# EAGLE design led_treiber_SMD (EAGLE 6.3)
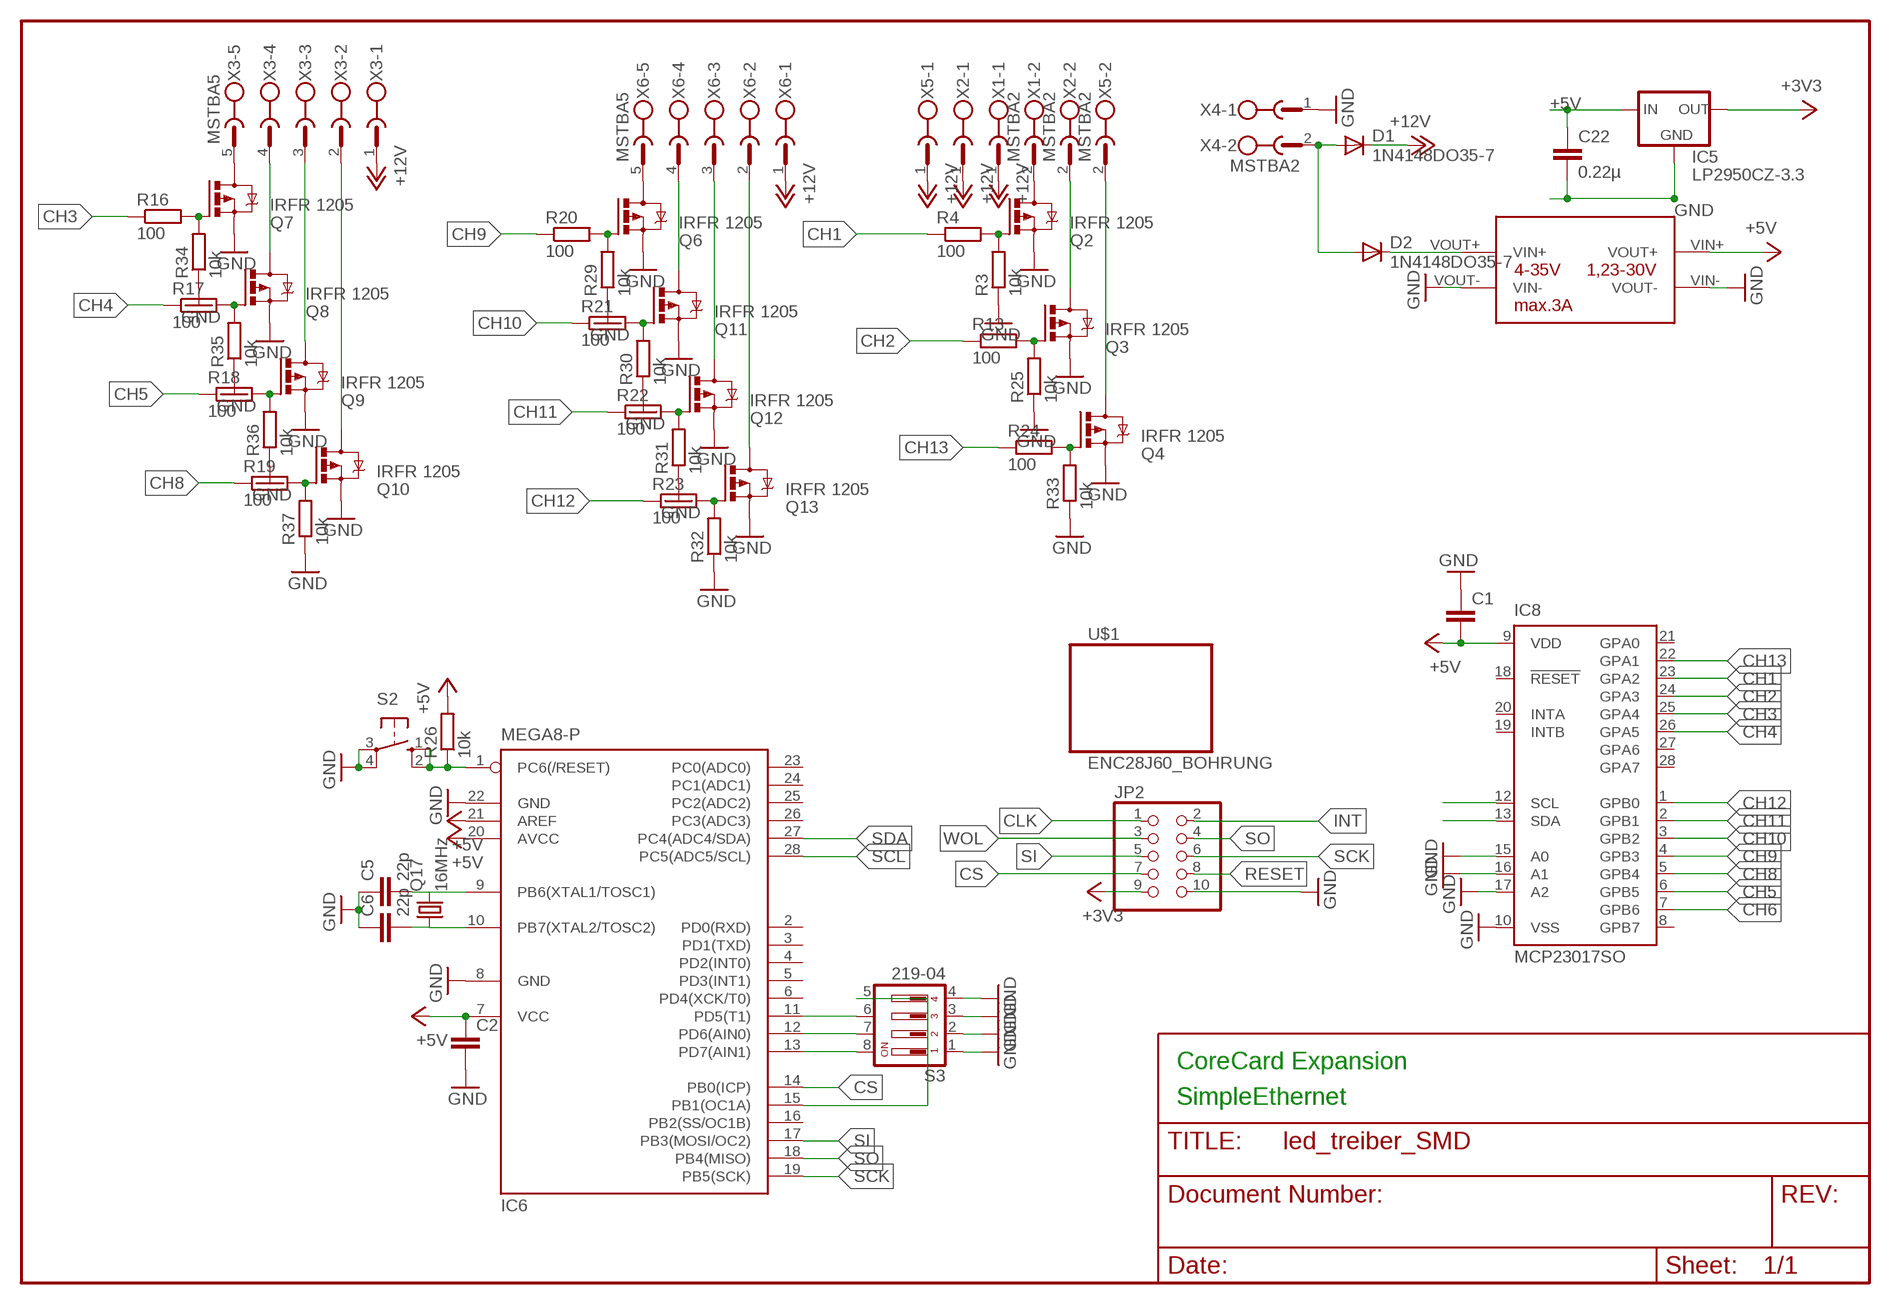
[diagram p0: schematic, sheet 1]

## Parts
C1  C-EUC0805  [C0805]
C2  C-EUC0805  [C0805]
C5  22p  C-EU025-025X050  [C025-025X050]
C6  22p  C-EU025-025X050  [C025-025X050]
C22  0.22µ  C-EUC0603  [C0603]
D1  1N4148DO35-7  [DO35-7]
D2  1N4148DO35-7  [DO35-7]
IC5  LP2950CZ-3.3  [TO92]
IC6  MEGA8-P  [DIL28-3]
IC8  MCP23017SO  [SO28W]
JP2  PINHD-2X5  [2X05]
Q2  IRFR 1205  IRFR5305  [D-PAK_TO252AA]
Q3  IRFR 1205  IRFR5305  [D-PAK_TO252AA]
Q4  IRFR 1205  IRFR5305  [D-PAK_TO252AA]
Q6  IRFR 1205  IRFR5305  [D-PAK_TO252AA]
Q7  IRFR 1205  IRFR5305  [D-PAK_TO252AA]
Q8  IRFR 1205  IRFR5305  [D-PAK_TO252AA]
Q9  IRFR 1205  IRFR5305  [D-PAK_TO252AA]
Q10  IRFR 1205  IRFR5305  [D-PAK_TO252AA]
Q11  IRFR 1205  IRFR5305  [D-PAK_TO252AA]
Q12  IRFR 1205  IRFR5305  [D-PAK_TO252AA]
Q13  IRFR 1205  IRFR5305  [D-PAK_TO252AA]
Q17  16MHz  CRYSTALHC49S  [HC49/S]
R3  10k  R-EU_M0805  [M0805]
R4  100  R-EU_R0805  [R0805]
R13  100  R-EU_M0805  [M0805]
R16  100  R-EU_M0805  [M0805]
R17  100  R-EU_M0805  [M0805]
R18  100  R-EU_M0805  [M0805]
R19  100  R-EU_M0805  [M0805]
R20  100  R-EU_R0805  [R0805]
R21  100  R-EU_R0805  [R0805]
R22  100  R-EU_R0805  [R0805]
R23  100  R-EU_M0805  [M0805]
R24  100  R-EU_M0805  [M0805]
R25  10k  R-EU_R0805  [R0805]
R26  10k  R-EU_M0805  [M0805]
R29  10k  R-EU_R0805  [R0805]
R30  10k  R-EU_R0805  [R0805]
R31  10k  R-EU_R0805  [R0805]
R32  10k  R-EU_M0805  [M0805]
R33  10k  R-EU_M0805  [M0805]
R34  10k  R-EU_M0805  [M0805]
R35  10k  R-EU_M0805  [M0805]
R36  10k  R-EU_M0805  [M0805]
R37  10k  R-EU_M0805  [M0805]
S2  10-XX  [B3F-10XX]
S3  219-04  [CTS-219-04]
U$1  ENC28J60_BOHRUNG  [ENC28J60_BOHRUNG]
U$2  SCHALTREGLER  [SCHALTREGLER_PLATINE]
X1  MSTBA2  [MSTBA2]
X2  MSTBA2  [MSTBA2]
X3  MSTBA5  [MSTBA5]
X4  MSTBA2  [MSTBA2]
X5  MSTBA2  [MSTBA2]
X6  MSTBA5  [MSTBA5]

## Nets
+3V3: IC5.1(OUT) JP2.9
+5V: C1.2 C2.1 C22.1 IC5.3(IN) IC6.7(VCC) IC6.20(AVCC) IC6.21(AREF) IC8.9(VDD) R26.2 U$2.VIN+(VOUT+)
+12V: D1.C X1.1 X2.1 X3.1 X5.1 X6.1
CH1: IC8.23(GPA2) R4.1
CH2: IC8.24(GPA3) R13.1
CH3: IC8.25(GPA4) R16.1
CH4: IC8.26(GPA5) R17.1
CH5: IC8.6(GPB5) R18.1
CH6: IC8.7(GPB6)
CH8: IC8.5(GPB4) R19.1
CH9: IC8.4(GPB3) R20.1
CH10: IC8.3(GPB2) R21.1
CH11: IC8.2(GPB1) R22.1
CH12: IC8.1(GPB0) R23.1
CH13: IC8.22(GPA1) R24.1
CLK: JP2.1
CS: IC6.14(PB0(ICP)) JP2.7
GND: C1.1 C2.2 C5.1 C6.1 C22.2 IC5.2(GND) IC6.8(GND) IC6.22(GND) IC8.10(VSS) IC8.15(A0) IC8.16(A1) IC8.17(A2) JP2.10 Q2.3(S) Q3.3(S) Q4.3(S) Q6.3(S) Q7.3(S) Q8.3(S) Q9.3(S) Q10.3(S) Q11.3(S) Q12.3(S) Q13.3(S) R3.1 R25.1 R29.1 R30.1 R31.1 R32.1 R33.1 R34.1 R35.1 R36.1 R37.1 S2.3(P) S2.4(P1) S3.1 S3.2 S3.3 S3.4 U$2.VIN-(VOUT-) U$2.VOUT-(VIN-) X4.1
INT: JP2.2
N$8: Q2.4(D) X1.2
N$11: Q6.4(D) X6.5
N$12: Q7.4(D) X3.5
N$15: Q2.1(G) R3.2 R4.2
N$19: Q3.1(G) R13.2 R25.2
N$20: Q4.4(D) X5.2
N$21: IC6.15(PB1(OC1A)) S3.5
N$22: Q7.1(G) R16.2 R34.2
N$23: Q8.1(G) R17.2 R35.2
N$24: Q9.1(G) R18.2 R36.2
N$25: Q10.1(G) R19.2 R37.2
N$26: Q6.1(G) R20.2 R29.2
N$27: Q11.1(G) R21.2 R30.2
N$28: Q12.1(G) R22.2 R31.2
N$29: Q13.1(G) R23.2 R32.2
N$30: Q4.1(G) R24.2 R33.2
N$31: D1.A D2.A X4.2
N$32: C5.2 IC6.9(PB6(XTAL1/TOSC1)) Q17.2
N$33: C6.2 IC6.10(PB7(XTAL2/TOSC2)) Q17.1
N$34: D2.C U$2.VOUT+(VIN+)
N$36: IC6.11(PD5(T1)) S3.6
N$37: IC6.12(PD6(AIN0)) S3.7
N$38: Q3.4(D) X2.2
N$41: IC6.13(PD7(AIN1)) S3.8
N$42: Q8.4(D) X3.4
N$43: Q9.4(D) X3.3
N$44: Q10.4(D) X3.2
N$46: Q11.4(D) X6.4
N$47: Q12.4(D) X6.3
N$48: Q13.4(D) X6.2
RESET: IC6.1(PC6(/RESET)) JP2.8 R26.1 S2.1(S) S2.2(S1)
SCK: IC6.19(PB5(SCK)) JP2.6
SCL: IC6.28(PC5(ADC5/SCL)) IC8.12(SCL)
SDA: IC6.27(PC4(ADC4/SDA)) IC8.13(SDA)
SI: IC6.17(PB3(MOSI/OC2)) JP2.5
SO: IC6.18(PB4(MISO)) JP2.4
WOL: JP2.3
Unconnected: IC6.2(PD0(RXD)) IC6.3(PD1(TXD)) IC6.4(PD2(INT0)) IC6.5(PD3(INT1)) IC6.6(PD4(XCK/T0)) IC6.16(PB2(SS/OC1B)) IC6.23(PC0(ADC0)) IC6.24(PC1(ADC1)) IC6.25(PC2(ADC2)) IC6.26(PC3(ADC3)) IC8.8(GPB7) IC8.18(!RESET) IC8.19(INTB) IC8.20(INTA) IC8.21(GPA0) IC8.27(GPA6) IC8.28(GPA7)

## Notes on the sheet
- CoreCard Expansion
- SimpleEthernet

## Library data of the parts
C1 C2 C5 C6 C22 = rcl:C-EU: CAPACITOR, European symbol
D1 D2 = diode:1N4148: DIODE
IC5 = v-reg:LP2950?*: Source: http://cache.national.com/ds/LP/LP2950.pdf
IC6 = atmel:MEGA8-P: MICROCONTROLLER 8 Kbytes FLASH, 1 kbytes SRAM, 512 bytes EEPROM, USART, 4-channel 10 bit ADC, 2-channel 8 bit ADC Pin compatible with Atmega48, ATMega88, ATMega168 Source: avr.lbr; OC_FARNELL: unknown; OC_NEWARK: unknown
IC8 = microchip:MCP23017: http://ww1.microchip.com/downloads/en/DeviceDoc/21952a.pdf Source: http://ww1.microchip.com/downloads/en/DeviceDoc/21952a.pdf; MF: MICROCHIP; MPN: MCP23017-E/SO; OC_FARNELL: 1332087; OC_NEWARK: 31K2958
JP2 = pinhead:PINHD-2X5: PIN HEADER
Q2-Q4 Q6-Q13 = transistor-power:IRF?5305: HEXFET Power MOSFET Source: http://www.irf.com/product-info/datasheets/data/irfr5305pbf.pdf
Q17 = crystal:CRYSTAL: CRYSTAL; OC_FARNELL: 1667008; OC_NEWARK: unknown
R3 R4 R13 R16-R26 R29-R37 = rcl:R-EU_: RESISTOR, European symbol
S2 = switch-omron:10-XX: OMRON SWITCH; MPN: B3F-1000; OC_FARNELL: 176432; OC_NEWARK: 36M3542
S3 = switch-dil:219-04*: Surface Mount DIP Switch Series 219 SMT CTS Electronic Components Sourc: www.ctscorp.com; OC_FARNELL: unknown; OC_NEWARK: unknown
U$1 = daniel:ENC28J60_BOHRUNG
U$2 = daniel:SCHALTREGLER
X1 X2 X4 X5 = con-phoenix-508:MSTBA2: PHOENIX; MF: FARNELL; MPN: 1757242; OC_FARNELL: 3705171; OC_NEWARK: 71C4161
X3 X6 = con-phoenix-508:MSTBA5: PHOENIX; MPN: 1757271; OC_FARNELL: 3705201; OC_NEWARK: 71C4164

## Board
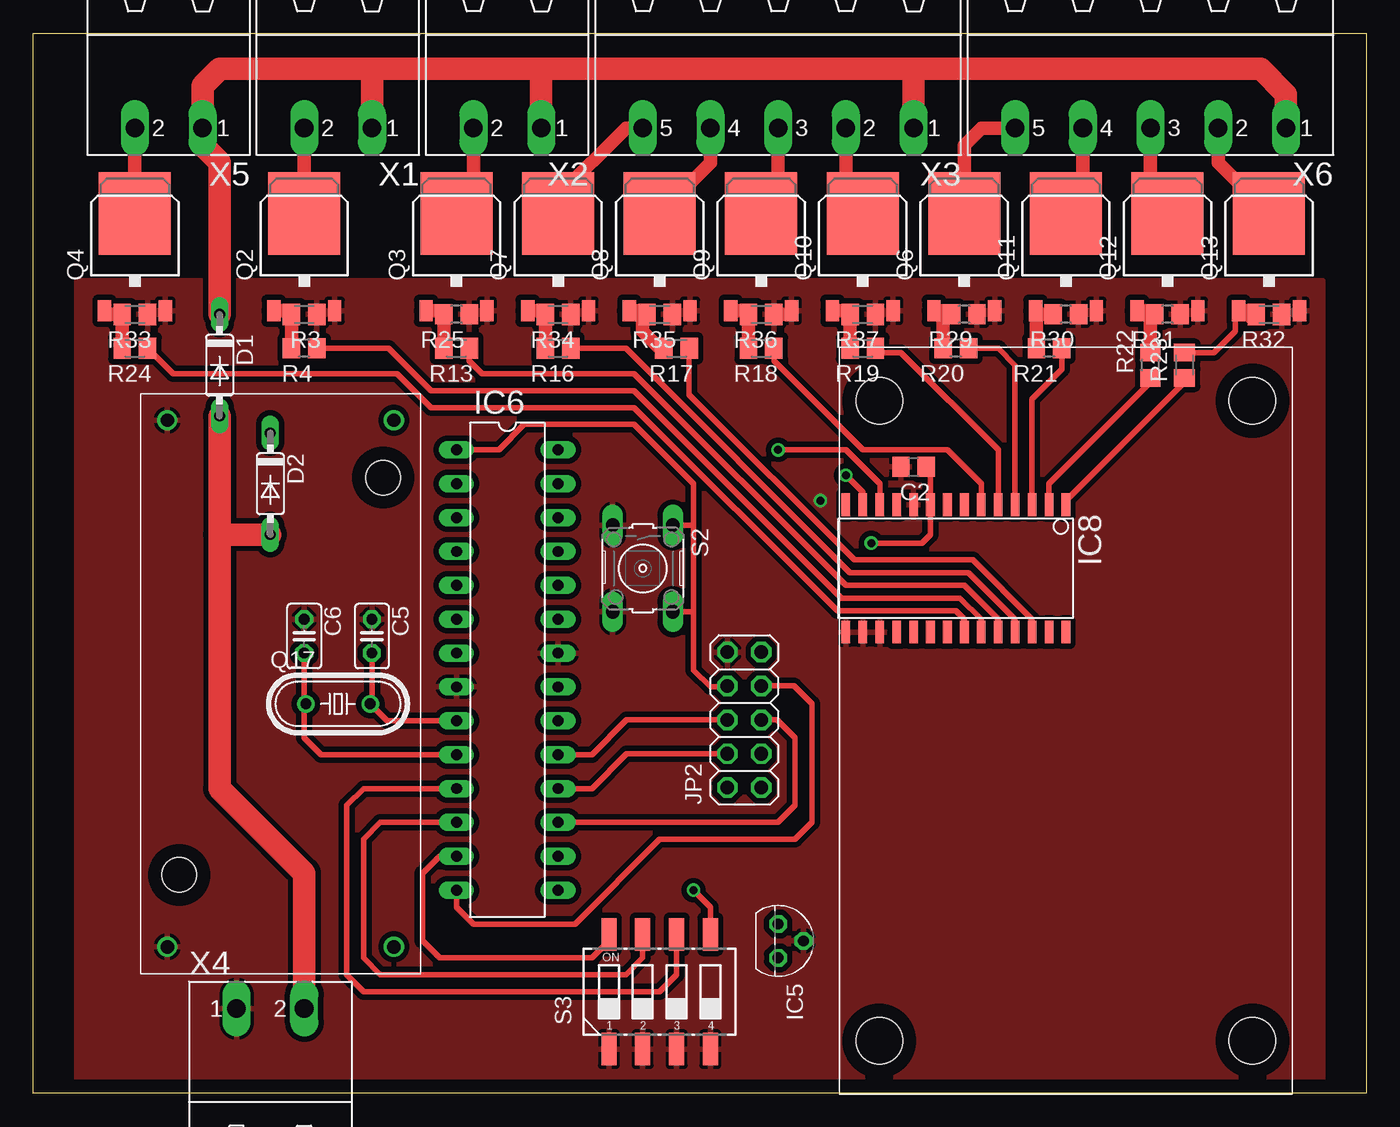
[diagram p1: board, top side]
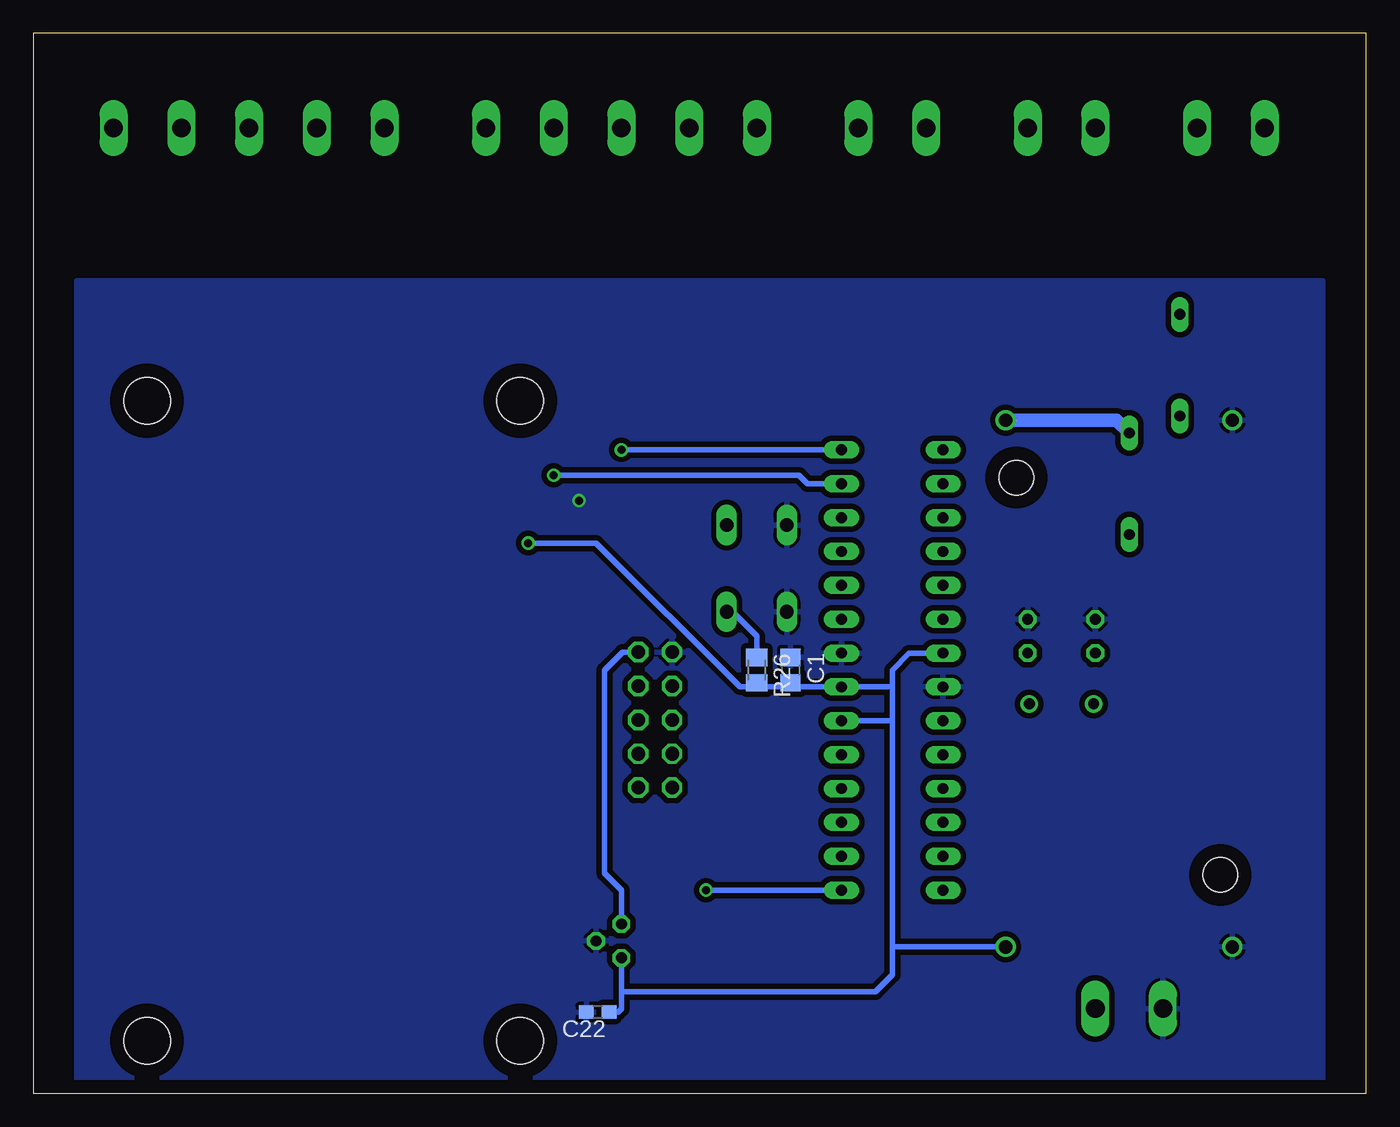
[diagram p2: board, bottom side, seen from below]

Size 100 x 79.5 mm. Coordinates in mm from the lower left corner, seen from the top.
Outline: 0,0 0,79.5 100,79.5 100,0 0,0
Copper layers (1*16): Top 0.035mm / dielectric 1.5mm / Bottom 0.035mm
Design rules "Bilex DRU": minimum track width 10mil, minimum drill 24mil, track to track 10mil, track to pad 10mil, pad to pad 10mil, via to via 10mil, smd to smd 10mil, copper to edge 40mil, drill to drill 8mil, minimum pad ring 10mil, minimum via ring 8mil, stop-mask expansion 4mil, vias tented up to drill 0mil, thermal gap 10mil

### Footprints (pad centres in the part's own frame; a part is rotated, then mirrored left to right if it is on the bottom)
C0805 = smd 1.3 x 1.5: 1 -0.95,0; 2 0.95,0
C025-025X050 = drill 0.813 octagon: 1 -1.27,0; 2 1.27,0
C0603 = smd 1.1 x 1: 1 -0.85,0; 2 0.85,0
DO35-7 = drill 0.813 long: A 3.81,0; C -3.81,0
TO92 = drill 0.813 octagon: 1 -1.27,0; 2 0,1.905; 3 1.27,0
DIL28-3 = drill 0.813 long: 1 -16.51,-3.81; 2 -13.97,-3.81; 3 -11.43,-3.81; 4 -8.89,-3.81; 5 -6.35,-3.81; 6 -3.81,-3.81; 7 -1.27,-3.81; 8 1.27,-3.81; 9 3.81,-3.81; 10 6.35,-3.81; 11 8.89,-3.81; 12 11.43,-3.81; 13 13.97,-3.81; 14 16.51,-3.81; 15 16.51,3.81; 16 13.97,3.81; 17 11.43,3.81; 18 8.89,3.81; 19 6.35,3.81; 20 3.81,3.81; 21 1.27,3.81; 22 -1.27,3.81; 23 -3.81,3.81; 24 -6.35,3.81; 25 -8.89,3.81; 26 -11.43,3.81; 27 -13.97,3.81; 28 -16.51,3.81
SO28W = smd 0.65 x 1.7: 1 -7.62,-4.78; 2 -6.35,-4.78; 3 -5.08,-4.78; 4 -3.81,-4.78; 5 -2.54,-4.78; 6 -1.27,-4.78; 7 0,-4.78; 8 1.27,-4.78; 9 2.54,-4.78; 10 3.81,-4.78; 11 5.08,-4.78; 12 6.35,-4.78; 13 7.62,-4.78; 14 8.89,-4.78; 15 8.89,4.78; 16 7.62,4.78; 17 6.35,4.78; 18 5.08,4.78; 19 3.81,4.78; 20 2.54,4.78; 21 1.27,4.78; 22 0,4.78; 23 -1.27,4.78; 24 -2.54,4.78; 25 -3.81,4.78; 26 -5.08,4.78; 27 -6.35,4.78; 28 -7.62,4.78
2X05 = drill 1.016 octagon: 1 -5.08,-1.27; 2 -5.08,1.27; 3 -2.54,-1.27; 4 -2.54,1.27; 5 0,-1.27; 6 0,1.27; 7 2.54,-1.27; 8 2.54,1.27; 9 5.08,-1.27; 10 5.08,1.27
D-PAK_TO252AA = smd 1 x 1.6: 1 -2.28,-4.8; 3 2.28,-4.8 | smd 5.4 x 6.2: 4 0,2.5
HC49/S = drill 0.813: 1 -2.413,0; 2 2.413,0
M0805 = smd 1.3 x 1.6: 1 -0.95,0; 2 0.95,0
R0805 = smd 1.3 x 1.5: 1 -0.95,0; 2 0.95,0
B3F-10XX = drill 1.016 long: 1 -3.251,2.261; 2 3.251,2.261; 3 -3.251,-2.261; 4 3.251,-2.261
CTS-219-04 = smd 1.13 x 2.44: 1 -3.81,-4.3; 2 -1.27,-4.3; 3 1.27,-4.3; 4 3.81,-4.3; 5 3.81,4.3; 6 1.27,4.3; 7 -1.27,4.3; 8 -3.81,4.3
ENC28J60_BOHRUNG = hole 3.5: -24,14; 24,-14; -24,-14; 24,14
SCHALTREGLER_PLATINE = drill 1: VIN+ 19.5,8; VIN- 19.5,-9; VOUT+ -20,8; VOUT- -20,-9 | hole 2.6: -15.7,7.2; 14.1,-8.1
MSTBA2 = drill 1.397 long: 1 -2.54,5.08; 2 2.54,5.08
MSTBA5 = drill 1.397 long: 1 -10.16,5.08; 2 -5.08,5.08; 3 0,5.08; 4 5.08,5.08; 5 10.16,5.08

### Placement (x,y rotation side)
C1  43.18,31.75 270 bottom
C2  66.04,46.99 180 top
C5  25.4,34.29 270 top
C6  20.32,34.29 270 top
C22  57.66,6.1 180 bottom
D1  13.97,54.61 270 top
D2  17.78,45.72 270 top
IC5  55.88,11.43 270 top
IC6  35.56,31.75 270 top
IC8  69.85,39.37 180 top
JP2  53.35,28.01 90 top
Q2  20.32,63.5 0 top
Q3  31.75,63.5 0 top
Q4  7.62,63.5 0 top
Q6  69.85,63.5 0 top
Q7  39.37,63.5 0 top
Q8  46.99,63.5 0 top
Q9  54.61,63.5 0 top
Q10  62.23,63.5 0 top
Q11  77.47,63.5 0 top
Q12  85.09,63.5 0 top
Q13  92.71,63.5 0 top
Q17  22.86,29.21 0 top
R3  20.32,58.42 180 top
R4  20.32,55.88 180 top
R13  31.75,55.88 180 top
R16  39.37,55.88 180 top
R17  48.26,55.88 180 top
R18  54.61,55.88 180 top
R19  62.23,55.88 180 top
R20  69.22,55.88 180 top
R21  76.2,55.88 180 top
R22  83.82,54.61 90 top
R23  86.36,54.61 90 top
R24  7.62,55.88 180 top
R25  31.75,58.42 180 top
R26  45.72,31.75 270 bottom
R29  69.85,58.42 180 top
R30  77.47,58.42 180 top
R31  85.09,58.42 180 top
R32  92.71,58.42 180 top
R33  7.62,58.42 180 top
R34  39.37,58.42 180 top
R35  46.99,58.42 180 top
R36  54.61,58.42 180 top
R37  62.23,58.42 180 top
S2  45.72,39.37 270 top
S3  46.99,7.62 0 top
U$1  77.47,27.94 90 top
U$2  19.05,30.48 270 top
X1  22.86,77.47 180 top
X2  35.56,77.47 180 top
X3  55.88,77.47 180 top
X4  17.78,1.27 0 top
X5  10.16,77.47 180 top
X6  83.82,77.47 180 top

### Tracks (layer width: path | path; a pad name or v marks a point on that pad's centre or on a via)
+3V3
  Bottom 0.406: JP2.9 55.81,33.09 57.15,31.75 57.15,16.51 55.88,15.24 IC5.1
+5V  (via drill 0.6)
  Top 0.406: C2.1 67.31,46.67 IC8.9 67.31,41.91 66.67,41.27 v62.87,41.27
  Bottom 0.406: 35.56,30.48 IC6.21 42.86,30.48 C1.2 43.5,30.48 45.72,30.48 | IC6.20 35.56,27.94 | 55.88,7.62 36.83,7.62 35.56,8.89 35.56,10.98 | C22.1 56.13,6.1 55.88,6.35 55.88,7.62 | 55.88,7.62 IC5.3 | 45.72,30.48 R26.2 | 45.72,30.48 46.99,30.48 57.78,41.27 v62.87,41.27 | 35.56,27.94 35.56,13.97 35.56,10.98 | 35.56,30.48 35.56,27.94 | IC6.7 34.29,33.02 35.56,31.75 35.56,30.48 | U$2.VIN+ 35.56,10.98
+12V
  Top 1.676: 25.4,76.83 13.97,76.83 12.7,75.56 X5.1 12.7,71.12 13.97,69.85 D1.C | 25.4,76.83 38.1,76.83 | 38.1,76.83 66.04,76.83 | 66.04,76.83 92.08,76.83 93.98,74.93 X6.1 | X3.1 66.04,76.83 | X2.1 38.1,76.83 | X1.1 25.4,76.83
CH1
  Top 0.406: IC8.23 71.12,35.56 69.53,37.15 60.64,37.15 45.09,52.7 29.84,52.7 26.67,55.88 R4.1
CH2
  Top 0.406: R13.1 32.7,54.93 33.66,53.98 45.09,53.98 60.96,38.1 69.85,38.1 72.39,35.56 IC8.24
CH3
  Top 0.406: IC8.25 73.66,35.56 70.17,39.05 61.28,39.05 44.45,55.88 R16.1
CH4
  Top 0.406: IC8.26 74.93,35.56 70.48,40.01 61.59,40.01 49.21,52.39 R17.1
CH5
  Top 0.406: R18.1 55.56,54.93 62.23,48.26 68.58,48.26 71.12,45.72 IC8.6
CH8
  Top 0.406: R19.1 63.5,55.56 65.09,55.56 72.39,48.26 IC8.5
CH9
  Top 0.406: IC8.4 73.66,54.61 72.39,55.88 R20.1
CH10
  Top 0.406: IC8.3 74.93,52.07 77.15,54.29 R21.1
CH11
  Top 0.406: 84.14,53.66 R22.1 83.82,53.34 76.2,45.72 IC8.2
CH12
  Top 0.406: IC8.1 77.47,44.45 86.36,53.34 R23.1
CH13
  Top 0.406: IC8.22 69.85,35.56 69.22,36.2 60.33,36.2 45.09,51.44 29.84,51.44 27.3,53.98 10.47,53.98 R24.1
CS
  Top 0.406: IC6.14 31.75,13.97 33.02,12.7 40.64,12.7 46.99,19.05 57.15,19.05 58.42,20.32 58.42,29.21 57.08,30.55 JP2.7
GND  (via drill 0.6)
  Top 0.406: IC8.15 60.96,34.09
  Top 1.016: R36.1 56.61,58.42 Q9.3
  other vias: 59.05,44.45
  pour Bottom (isolate 0.406): 3.27,60.96 96.73,60.96 96.73,0 3.27,0
  pour Top (isolate 0.406): 3.27,60.96 96.73,60.96 96.73,0 3.27,0
N$8
  Top 1.016: X1.2 Q2.4
N$11
  Top 1.016: X6.5 71.12,72.39 69.85,71.12 Q6.4
N$12
  Top 1.016: X3.5 44.45,72.39 39.37,67.31 Q7.4
N$15
  Top 1.016: R4.2 R3.2 19.09,58.7 Q2.1
N$19
  Top 1.016: R13.2 R25.2 30.52,58.7 Q3.1
N$20
  Top 1.016: X5.2 Q4.4
N$21  (via drill 0.6)
  Top 0.406: S3.5 50.8,13.97 v49.53,15.24
  Bottom 0.406: IC6.15 v49.53,15.24
N$22
  Top 1.016: R16.2 R34.2 38.14,58.7 Q7.1
N$23
  Top 1.016: R17.2 46.99,55.88 45.72,57.15 45.72,58.1 R35.2 45.76,58.7 Q8.1
N$24
  Top 1.016: R18.2 R36.2 53.38,58.7 Q9.1
N$25
  Top 1.016: Q10.1 61,58.7 R37.2 R19.2
N$26
  Top 1.016: R20.2 68.26,58.1 68.58,58.42 R29.2 68.62,58.7 Q6.1
N$27
  Top 1.016: R21.2 75.25,58.64 Q11.1 75.47,58.42 R30.2
N$28
  Top 1.016: R22.2 83.82,58.1 R31.2 83.86,58.7 Q12.1
N$29
  Top 0.406: R23.2 88.58,55.56 90.17,57.15 90.17,58.44 Q13.1
  Top 1.016: Q13.1 91.48,58.7 R32.2 91.44,58.1
N$30
  Top 1.016: Q4.1 5.62,58.42 R33.2 R24.2
N$31
  Top 1.676: D1.A 13.97,41.91 | 13.97,41.91 13.97,22.86 20.32,16.51 X4.2 | D2.A 13.97,41.91
N$32
  Top 0.406: IC6.9 26.54,27.94 Q17.2 25.4,29.34 C5.2
N$33
  Top 0.406: IC6.10 21.59,25.4 20.32,26.67 20.32,29.08 Q17.1 20.32,29.34 C6.2
N$34
  Bottom 1.016: U$2.VOUT+ 18.73,50.48 D2.C
N$36
  Top 0.406: IC6.11 24.77,22.86 23.5,21.59 23.5,8.89 24.77,7.62 46.99,7.62 48.26,8.89 S3.6
N$37
  Top 0.406: IC6.12 26.04,20.32 24.77,19.05 24.77,10.16 26.04,8.89 44.45,8.89 45.72,10.16 S3.7
N$38
  Top 1.016: X2.2 33.02,67.27 Q3.4
N$41
  Top 0.406: IC6.13 30.48,17.78 29.21,16.51 29.21,11.43 30.48,10.16 41.91,10.16 43.18,11.43 S3.8
N$42
  Top 1.016: X3.4 50.8,69.81 Q8.4
N$43
  Top 1.016: X3.3 55.88,67.27 Q9.4
N$44
  Top 1.016: X3.2 60.96,67.27 Q10.4
N$46
  Top 1.016: X6.4 78.74,67.27 Q11.4
N$47
  Top 1.016: X6.3 83.82,67.27 Q12.4
N$48
  Top 1.016: X6.2 88.9,69.81 Q13.4
RESET
  Top 0.406: IC6.1 34.92,48.26 36.83,50.16 45.09,50.16 49.53,45.72 49.53,42.55 | 49.53,42.55 49.53,36.2 | 49.53,36.2 49.53,31.75 50.8,30.48 52.01,30.48 JP2.8 | S2.1 49.45,42.62 49.53,42.55 | S2.2 49.45,36.12 49.53,36.2
  Bottom 0.406: R26.1 45.72,34.29 47.55,36.12 S2.2
SCK
  Top 0.406: JP2.6 44.52,28.01 41.91,25.4 IC6.19
SCL  (via drill 0.6)
  Top 0.406: v55.88,48.26 60.96,48.26 63.5,45.72 IC8.12
  Bottom 0.406: IC6.28 v55.88,48.26
SDA  (via drill 0.6)
  Top 0.406: IC8.13 62.23,45.09 v60.96,46.35
  Bottom 0.406: v60.96,46.35 42.55,46.35 41.91,45.72 IC6.27
SI
  Top 0.406: JP2.5 55.81,28.01 57.15,26.67 57.15,21.59 55.88,20.32 IC6.17
SO
  Top 0.406: JP2.4 44.52,25.47 41.91,22.86 IC6.18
